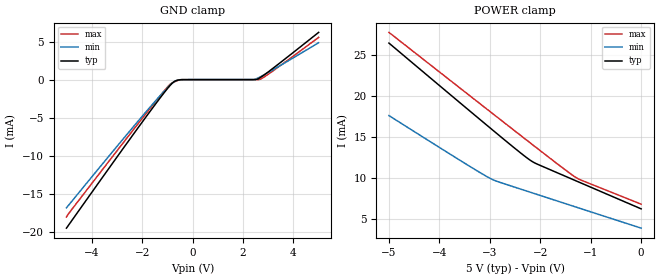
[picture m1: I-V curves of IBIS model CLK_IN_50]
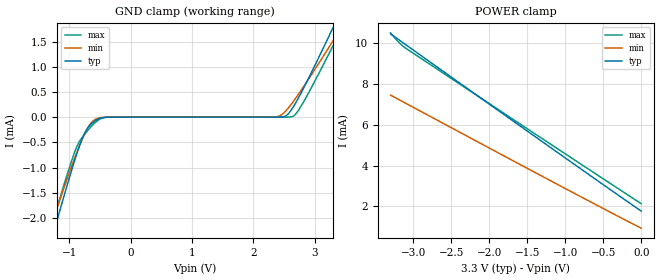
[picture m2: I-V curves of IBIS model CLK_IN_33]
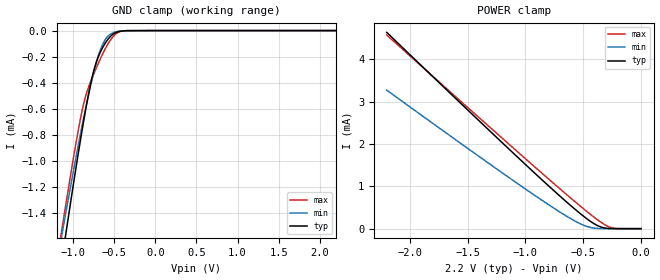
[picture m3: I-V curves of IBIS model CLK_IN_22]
| TEXAS INSTRUMENTS INCORPORATED
| Standard Linear and Logic Group
| IBIS Model of CDC3RL02
| Low Phase-Noise Two Channel Clock Fan-Out Buffer
| This file contains package information for the following:
|  WLBGA 8-pin (YEP_YZP) package as [Component] CDC3RL02_YEP_YZP
| This device can be powered at the following Vccs:
|  5 volt Vcc
|  3.3 volt Vcc
|  2.2 volt Vcc
| This file provides unique models under the [Model Selector] for each Vcc.
| For operation at a specific Vcc, select the appropriate model after each
| [Model Selector] keyword.
[IBIS Ver]   3.2
[Comment char]  |_char
[File Name]   cdc3rl02.ibs
[File Rev]   1 | A1
[Date]   April 8, 2011
[Source]   Data created from TI-SPICE simulations at TI-SLL.
[Notes]   The following is an IBIS list for the CDC3RL02.
   Please contact sllibis@ti.com with questions and
   comments concerning SLL IBIS models.
   A load capacitor of 30pF on the CLK_OUTx pins has been
   built into the IBIS model to capture effect of output
   buffer slew control.
   Power-clamp waveforms for MCLK_IN pin does not cross zero
   at the 5.0V and 3.3V nodes due to since input range of this
   pin is restricted between GND and VLDO output regardless of
   VBAT supply.
[Disclaimer] Property of Texas Instruments Incorporated.  Unauthorized
   reproduction and/or distribution is strictly prohibited.
   This product is protected under copyright law.
   Created  2011, (C) Copyright  2011, Texas Instruments
   Incorporated, All Rights Reserved
   UNLESS THERE IS A SIGNED, WRITTEN AGREEMENT TO THE
   CONTRARY, TEXAS INSTRUMENTS (TI) IS PROVIDING THE IBIS
   MODELS  AND WITHOUT ANY WARRANTY, EXPRESSED OR
   IMPLIED.  TI assumes no liability for:
   1) the accuracy of the IBIS models provided to your
   company;
   2) the proper functioning of these IBIS Models in your
   design or for any resulting applications; or
   3) infringement of patents, copyrights or intellectual
   property rights resulting from your use of these IBIS
   models.
   TI provides IBIS Models as a service to our customers.
   You and your company shall not distribute, sell or give
   these models to anyone else without prior written
   permission from TI.
   TI reserves the right to make changes to our products or
   to discontinue any semiconductor product or service
   without notice, and advises our customers to obtain the
   latest version of relevant information to verify, before
   placing orders, that the information being relied on is
   current.
   Please be aware that your receipt and use of the IBIS
   information provided shall serve as acceptance of these
   terms and conditions.  If you do not accept these terms,
   you should return or destroy the IBIS models and any
   other accompanying information immediately.
| Component CDC3RL02_YEP_YZP 8-PIN WLBGA
[Component]   CDC3RL02_YEP_YZP
[Manufacturer]   Texas Instruments, Inc.
[Package]
|   typ   min   max
R_pkg   1.000e-03   1.000e-03   4.000e-03
L_pkg   6.400e-11   2.400e-11   3.790e-10
C_pkg   5.800e-14   0.000e+00   6.700e-14
[Pin]   signal_name   model_name   R_pin   L_pin   C_pin
A1   VBATT   POWER   1.000e-03   2.500e-11   6.400e-14
B1   VLDO   POWER   1.000e-03   2.400e-11   6.700e-14
C1   MCLK_IN   CLK_IN   1.000e-03   2.400e-11   6.700e-14
D1   GND   GND   1.000e-03   2.500e-11   6.400e-14
A2   CLK_OUT1   CLK_OUT   1.000e-03   2.500e-11   6.400e-14
B2   CLK_REQ1   CLK_REQ   1.000e-03   2.400e-11   6.700e-14
C2   CLK_REQ2   CLK_REQ   1.000e-03   2.400e-11   6.700e-14
D2   CLK_OUT2   CLK_OUT   1.000e-03   2.500e-11   6.400e-14
| Model CLK_IN
[Model Selector]   CLK_IN
CLK_IN_50   5 volt Vcc
CLK_IN_33   3.3 volt Vcc
CLK_IN_22   2.2 volt Vcc
| Model CLK_REQ
[Model Selector]   CLK_REQ
CLK_REQ_50   5 volt Vcc
CLK_REQ_33   3.3 volt Vcc
CLK_REQ_22   2.2 volt Vcc
| Model CLK_OUT
[Model Selector]   CLK_OUT
CLK_OUT_50   5 volt Vcc
CLK_OUT_33   3.3 volt Vcc
CLK_OUT_22   2.2 volt Vcc
| Models and submodels in the file (9): CLK_IN_50 (Input), CLK_IN_33 (Input), CLK_IN_22 (Input), CLK_REQ_50 (Input), CLK_REQ_33 (Input), CLK_REQ_22 (Input), CLK_OUT_50 (Output), CLK_OUT_33 (Output), CLK_OUT_22 (Output)
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[Model]   CLK_IN_50
Model_type  Input
Vinl=0.5
Vinh=1.3
| variable   typ   min   max
C_comp   3.55pF   2.48pF   4.21pF
[Temperature Range]   40   100   -40
| Ambient temperature   25   85   -40
[Voltage range]   5   4.5   5.5
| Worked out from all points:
|   GND clamp passes 1 mA (typ) near -0.95 V on its own axis
[GND Clamp]
| CLK_IN_50
|   Voltage   I(typ)   I(min)   I(max)
-5V       -19.55mA   -16.88mA   -18.08mA
-2.905V   -9.77mA    -8.423mA   -8.984mA
-1.555V   -3.601mA   -3.127mA   -3.253mA
-970mV    -1.078mA   -993.3uA   -885.9uA
-760mV    -339uA     -352.7uA   -351.7uA
-610mV    -98.47uA   -71.01uA   -142.6uA
-400mV    -3.032uA   -2.117uA   -3.859uA
2.335V    27.97nA    1.899uA    27.87pA
2.56V     52.41uA    163.7uA    310.2nA
2.7V      299.5uA    389.3uA    72.85uA
2.94V     863.4uA    824.1uA    565.3uA
5V        6.219mA    4.86mA     5.56mA
[POWER Clamp]
| CLK_IN_50
|   Voltage   I(typ)   I(min)   I(max)
-5V       26.44mA    17.59mA    27.74mA
-3.585V   19.12mA    12.12mA    20.92mA
-3.02V    16.22mA    10.03mA    18.2mA
-2.85V    15.35mA    9.558mA    17.39mA
-2.18V    12.07mA    8.212mA    14.17mA
-2.065V   11.69mA    7.982mA    13.62mA
-1.5V     10.19mA    6.853mA    10.95mA
-1.26V    9.552mA    6.374mA    9.926mA
-84.45fV  6.219mA    3.867mA    6.79mA
[Model]   CLK_IN_33
Model_type  Input
Vinl=0.5
Vinh=1.3
| variable   typ   min   max
C_comp   3.61pF   2.51pF   4.22pF
[Temperature Range]   40   100   -40
| Ambient temperature   25   85   -40
[Voltage range]   3.3   3   3.6
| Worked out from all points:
|   GND clamp passes 1 mA (typ) near -0.95 V on its own axis
[GND Clamp]
| CLK_IN_33
|   Voltage   I(typ)   I(min)   I(max)
-3.3V     -11.6mA    -10mA      -10.68mA
-1.335V   -2.626mA   -2.298mA   -2.338mA
-1.25V    -2.256mA   -1.984mA   -1.989mA
-925mV    -900.2uA   -844.5uA   -727.3uA
-780mV    -393.4uA   -405.9uA   -382.8uA
-630mV    -119.6uA   -93.09uA   -167.4uA
-475mV    -14.16uA   -8.784uA   -23.45uA
2.32V     16.2nA     1.209uA    25.23pA
2.53V     25.31uA    122.3uA    70.84nA
2.645V    186.9uA    296.3uA    15.23uA
2.735V    376.4uA    450.3uA    130.4uA
3.3V      1.772mA    1.51mA     1.412mA
[POWER Clamp]
| CLK_IN_33
|   Voltage   I(typ)   I(min)   I(max)
-3.3V     10.45mA    7.452mA    10.5mA
-3.18V    10.13mA    7.213mA    9.997mA
-3.085V   9.883mA    7.023mA    9.712mA
-1.08V    4.586mA    3.037mA    4.774mA
-48.03fV  1.772mA    936.7uA    2.135mA
[Model]   CLK_IN_22
Model_type  Input
Vinl=0.5
Vinh=1.3
| variable   typ   min   max
C_comp   3.67pF   2.72pF   4.23pF
[Temperature Range]   40   100   -40
| Ambient temperature   25   85   -40
[Voltage range]   2.2   2   2.4
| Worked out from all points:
|   GND clamp passes 1 mA (typ) near -0.95 V on its own axis
|   POWER clamp passes 1 mA (typ) near -0.80 V on its own axis
[GND Clamp]
| CLK_IN_22
|   Voltage   I(typ)   I(min)   I(max)
-2.2V     -6.523mA   -5.628mA   -5.975mA
-1.155V   -1.847mA   -1.639mA   -1.604mA
-1.125V   -1.719mA   -1.531mA   -1.484mA
-1.1V     -1.613mA   -1.442mA   -1.385mA
-1.075V   -1.508mA   -1.354mA   -1.286mA
-895mV    -785.4uA   -748uA     -630.9uA
-835mV    -568.2uA   -562.9uA   -478.6uA
-765mV    -352uA     -365.8uA   -359.4uA
-645mV    -136.9uA   -113uA     -186.8uA
-530mV    -36.07uA   -22.03uA   -59.39uA
-340mV    -751.7nA   -624.6nA   -629.7nA
2.2V      391pA      30.91nA    21.37pA
[POWER Clamp]
| CLK_IN_22
|   Voltage   I(typ)   I(min)   I(max)
-2.2V     4.639mA    3.274mA    4.577mA
-1.44V    2.651mA    1.782mA    2.719mA
-945mV    1.377mA    833.4uA    1.52mA
-650mV    644.4uA    304.5uA    819.4uA
-490mV    278.2uA    74.24uA    452.4uA
-430mV    158.7uA    24.88uA    320.9uA
-370mV    64.26uA    5.299uA    196.6uA
-320mV    19.11uA    1.209uA    104.4uA
-265mV    3.165uA    225.4nA    30.26uA
-205mV    362.8nA    35.97nA    2.724uA
0V        0A         0A         0A
